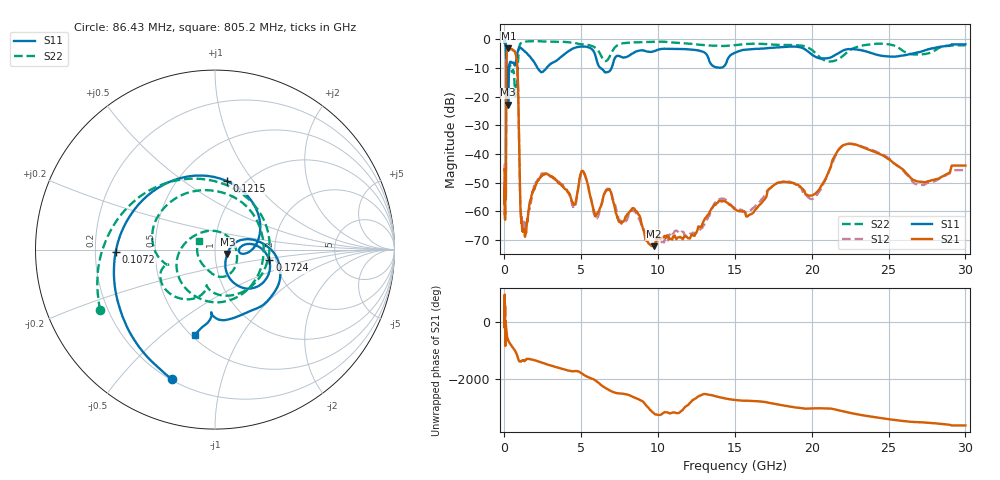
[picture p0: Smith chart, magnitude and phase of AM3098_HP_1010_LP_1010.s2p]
! Date/Time: Thu, Feb 28, 2019 8:42 AM
! Network Analyzer: Agilent Technologies E8364B Rev: A.07.50.67
! Sweep from 0.010 to 30.000 GHz, 1601 Points, Sweep Type: LOG
! Power Supply: 5.022 V, 0.002 A
# Hz S DB R 50
!freq MagS11 AngS11 MagS21 AngS21 MagS12 AngS12 MagS22 AngS22
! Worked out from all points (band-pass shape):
!   1601 points, 10 MHz to 30 GHz, reference 50 ohm
!   highest |S21| = -3.09 dB at 254.7 MHz (marker M1); lowest = -72.2 dB at 9.731 GHz (marker M2)
!   |S21| within 3 dB of the highest: 133.9 MHz to 771.5 MHz (637.7 MHz wide, 141 % of centre)
!   lowest |S11| = -22.7 dB at 241.1 MHz (marker M3), VSWR 1.16, Z = 57.3 - j2.75 ohm
!   |S11| at or under -10 dB: 191.7 MHz to 304.4 MHz (112.7 MHz wide, 45.4 % of centre); 2.155 GHz to 2.737 GHz (582 MHz wide, 23.8 % of centre); 6.264 GHz to 6.97 GHz (705.8 MHz wide, 10.7 % of centre)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
!   |S22| runs from -20.0 to -0.6 dB; largest |S21 - S12| = 0.01
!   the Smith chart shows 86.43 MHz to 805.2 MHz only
!   S11 on the Smith chart (normalised r, x): 86.43 MHz: 0.20, -0.70; 107.2 MHz: 0.29, -0.01; 121.5 MHz: 0.83, +0.75; 172.4 MHz: 1.85, -0.24; 805.2 MHz: 0.52, -0.65
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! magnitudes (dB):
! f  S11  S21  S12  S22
! 10 MHz  -0.3  -45.3  -43.8  -0.6
! 38.04 MHz  -0.4  -59.6  -61.0  -0.9
! 50.34 MHz  -0.7  -49.8  -48.2  -1.2
! 86.43 MHz  -2.4  -54.9  -55.2  -2.8
! 107.2 MHz  -5.1  -32.4  -31.8  -6.5
! 121.5 MHz  -8.2  -12.8  -12.8  -10.4
! 144.7 MHz  -17.5  -4.7  -4.6  -13.7
! 172.4 MHz  -10.2  -3.9  -3.9  -9.5
! 241.1 MHz  -22.7  -3.1  -3.1  -11.2
! 254.7 MHz  -19.3  -3.1  -3.0  -11.0
! 550.5 MHz  -8.0  -3.7  -3.7  -10.6
! 805.2 MHz  -6.2  -7.5  -7.5  -19.8
! 1.029 GHz  -2.9  -57.1  -56.5  -1.6
! 1.137 GHz  -3.3  -65.0  -63.7  -1.1
! 2.084 GHz  -9.3  -50.3  -50.0  -0.6
! 4.503 GHz  -3.0  -57.6  -58.9  -1.1
! 5.103 GHz  -2.4  -45.9  -46.0  -1.7
! 7.926 GHz  -6.1  -61.7  -63.3  -1.2
! 9.731 GHz  -4.1  -72.2  -68.2  -0.8
! 20.1 GHz  -5.6  -54.3  -55.6  -4.1
! 22.56 GHz  -3.3  -36.5  -36.4  -3.5
! 30 GHz  -1.7  -44.0  -45.7  -2.1
